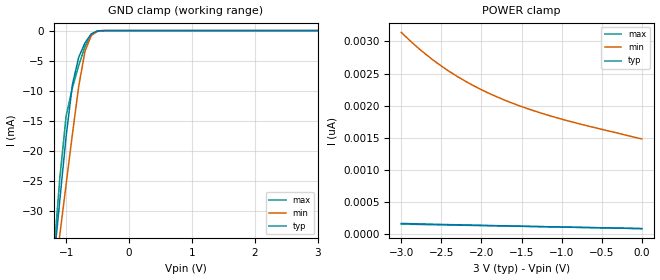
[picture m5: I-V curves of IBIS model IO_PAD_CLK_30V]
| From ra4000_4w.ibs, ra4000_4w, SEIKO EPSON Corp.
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[Model]   IO_PAD_CLK_30V
Model_type Input
Polarity Non-Inverting
Vinh=2.10
Vinl=0.90
C_comp   2.5p   2.0p   3.0p
[Temperature Range] 25   125   -40
[Voltage Range]   3.00   2.70   3.30
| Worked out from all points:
|   GND clamp passes 1 mA (typ) near -0.63 V on its own axis
[GND Clamp]
-3V       -236.1mA   -197.2mA   -285.1mA
-1.2V     -38.93mA   -42.41mA   -37.92mA
-1.1V     -28.21mA   -33.99mA   -24.54mA
-1V       -17.61mA   -25.59mA   -14.21mA
-900mV    -8.987mA   -17.22mA   -9.509mA
-800mV    -4.449mA   -9.275mA   -5.815mA
-700mV    -2.032mA   -3.425mA   -2.638mA
-600mV    -545.3uA   -804.5uA   -605.9uA
-500mV    -56.89uA   -135.5uA   -35.53uA
-400mV    -3.147uA   -16.88uA   -734nA
3V        88.04pA    1.573nA    80.87pA
[POWER Clamp]
-3V       169pA      3.14nA     158.9pA
-2.9V     165.9pA    3.02nA     156.6pA
-2.7V     159.8pA    2.804nA    152pA
-2.6V     156.8pA    2.707nA    149.7pA
-2.4V     151pA      2.532nA    145.1pA
-2.3V     148.1pA    2.453nA    142.8pA
-2.1V     142.6pA    2.312nA    138.2pA
-1.8V     134.4pA    2.133nA    131.3pA
-1.5V     126.5pA    1.986nA    124.4pA
-1.1V     116.3pA    1.827nA    115.2pA
-700mV    106.2pA    1.693nA    106pA
0V        88.04pA    1.484nA    89.13pA
